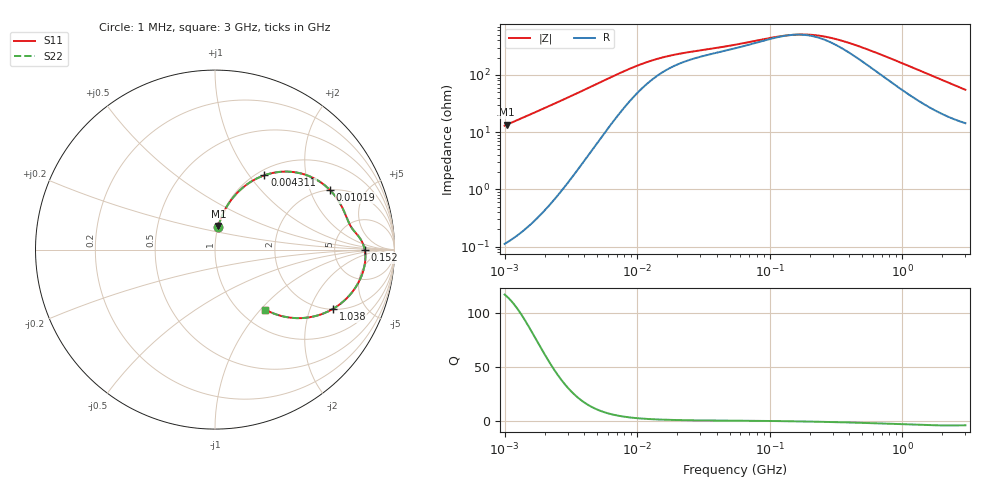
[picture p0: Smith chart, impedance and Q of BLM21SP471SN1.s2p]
! BLM21SP471SN1
# Hz S RI R 50
!Freq.(Hz) S11(Real) S11(Imag) S21(Real) S21(Imag) S12(Real) S12(Imag) S22(Real) S22(Imag)
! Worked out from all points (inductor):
!   401 points, 1 MHz to 3 GHz, reference 50 ohm
!   read as one part in series: L = 2.07 uH near 1.041 MHz
!   highest Q = 115 at 1.041 MHz (marker M1), where L = 2.06 uH
!   self-resonance near 150.2 MHz
!   S11 on the Smith chart (normalised r, x): 1 MHz: 1.00, +0.26; 4.311 MHz: 1.08, +1.19; 10.19 MHz: 2.00, +2.77; 152 MHz: 11, -0; 1.038 GHz: 2.03, -2.92; 3 GHz: 1.29, -1.06
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1000000  0.0176 0.1272  0.9824 -0.1272  0.9824 -0.1272  0.0176 0.1272
1040844  0.019 0.1322  0.981 -0.1322  0.981 -0.1322  0.019 0.1322
2226959  0.0838 0.2678  0.9162 -0.2678  0.9162 -0.2678  0.0838 0.2678
2947212  0.1425 0.3343  0.8575 -0.3343  0.8575 -0.3343  0.1425 0.3343
3823119  0.2263 0.393  0.7737 -0.393  0.7737 -0.393  0.2263 0.393
4310966  0.2754 0.4142  0.7246 -0.4142  0.7246 -0.4142  0.2754 0.4142
5266264  0.3685 0.4336  0.6315 -0.4336  0.6315 -0.4336  0.3685 0.4336
6433254  0.4664 0.4271  0.5336 -0.4271  0.5336 -0.4271  0.4664 0.4271
8179831  0.5705 0.3867  0.4295 -0.3867  0.4295 -0.3867  0.5705 0.3867
1.019448e7  0.6404 0.3319  0.3596 -0.3319  0.3596 -0.3319  0.6404 0.3319
1.461624e7  0.7044 0.2435  0.2956 -0.2435  0.2956 -0.2435  0.7044 0.2435
2.509235e7  0.743 0.1561  0.257 -0.1561  0.257 -0.1561  0.743 0.1561
5.477226e7  0.7844 0.0926  0.2156 -0.0926  0.2156 -0.0926  0.7844 0.0926
1.103592e8  0.8239 0.0336  0.1761 -0.0336  0.1761 -0.0336  0.8239 0.0336
1.520175e8  0.8344 -0.00143  0.1656 0.00143  0.1656 0.00143  0.8344 -0.00143
2.094008e8  0.8379 -0.0414  0.1621 0.0414  0.1621 0.0414  0.8379 -0.0414
3.453811e8  0.8267 -0.1158  0.1733 0.1158  0.1733 0.1158  0.8267 -0.1158
5.473095e8  0.7892 -0.201  0.2108 0.201  0.2108 0.201  0.7892 -0.201
8.005644e8  0.7249 -0.28  0.2751 0.28  0.2751 0.28  0.7249 -0.28
1.038491e9  0.6573 -0.3302  0.3427 0.3302  0.3427 0.3302  0.6573 -0.3302
1.747494e9  0.472 -0.3819  0.528 0.3819  0.528 0.3819  0.472 -0.3819
3e9  0.2805 -0.3342  0.7195 0.3342  0.7195 0.3342  0.2805 -0.3342
